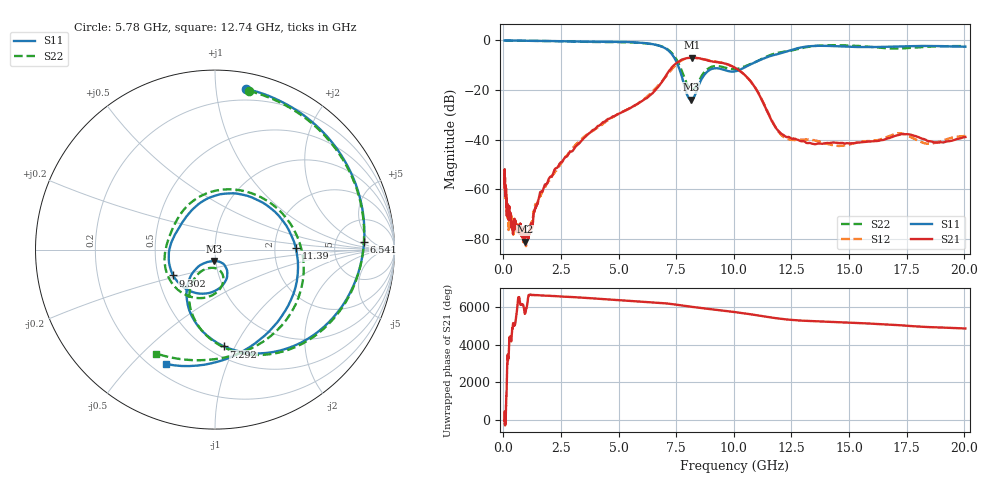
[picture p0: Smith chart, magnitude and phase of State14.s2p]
# Hz S DB R 50
!freq MagS11 AngS11 MagS21 AngS21 MagS12 AngS12 MagS22 AngS22
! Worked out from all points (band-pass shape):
!   1601 points, 50 MHz to 20.05 GHz, reference 50 ohm
!   highest |S21| = -6.96 dB at 8.19 GHz (marker M1); lowest = -81.3 dB at 929 MHz (marker M2)
!   |S21| within 3 dB of the highest: 7.409 GHz to 9.824 GHz (2.415 GHz wide, 28 % of centre)
!   lowest |S11| = -23.9 dB at 8.129 GHz (marker M3), VSWR 1.14, Z = 49.2 - j6.32 ohm
!   |S11| at or under -10 dB: 7.573 GHz to 10.65 GHz (3.077 GHz wide, 33.8 % of centre)
!   |S22| runs from -19.8 to 0.0 dB; largest |S21 - S12| = 0.026
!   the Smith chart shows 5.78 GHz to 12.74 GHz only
!   S11 on the Smith chart (normalised r, x): 5.78 GHz: 0.11, +1.20; 6.541 GHz: 10, +3; 7.292 GHz: 0.59, -0.90; 9.302 GHz: 0.60, -0.19; 11.39 GHz: 2.64, +0.05; 12.74 GHz: 0.26, -0.63
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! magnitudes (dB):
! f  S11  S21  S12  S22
! 50 MHz  0.0  -59.4  -53.9  0.0
! 53.69 MHz  0.0  -52.0  -55.1  0.0
! 72.72 MHz  0.0  -62.3  -61.1  0.0
! 99.62 MHz  0.0  -59.5  -61.9  0.0
! 135.9 MHz  0.0  -66.5  -66.5  0.0
! 217.1 MHz  0.0  -71.8  -73.6  0.0
! 248.5 MHz  0.0  -67.7  -71.5  0.0
! 369.6 MHz  0.0  -75.1  -74.7  0.0
! 929 MHz  -0.1  -81.3  -81.0  -0.1
! 1.005 GHz  -0.1  -78.4  -80.1  -0.1
! 2.722 GHz  -0.3  -47.0  -46.8  -0.4
! 5.78 GHz  -0.8  -25.8  -25.8  -0.9
! 6.541 GHz  -1.6  -20.6  -19.9  -1.6
! 7.292 GHz  -5.3  -11.0  -11.8  -4.9
! 7.402 GHz  -6.8  -10.0  -10.6  -6.2
! 8.129 GHz  -23.9  -7.0  -7.0  -19.7
! 8.19 GHz  -23.7  -7.0  -7.0  -19.8
! 9.302 GHz  -11.2  -8.8  -8.7  -10.3
! 10.45 GHz  -11.0  -13.7  -13.7  -10.6
! 11.39 GHz  -6.9  -27.5  -27.2  -6.7
! 12.74 GHz  -3.2  -40.0  -40.2  -3.5
! 20.05 GHz  -2.5  -39.0  -38.6  -2.3
